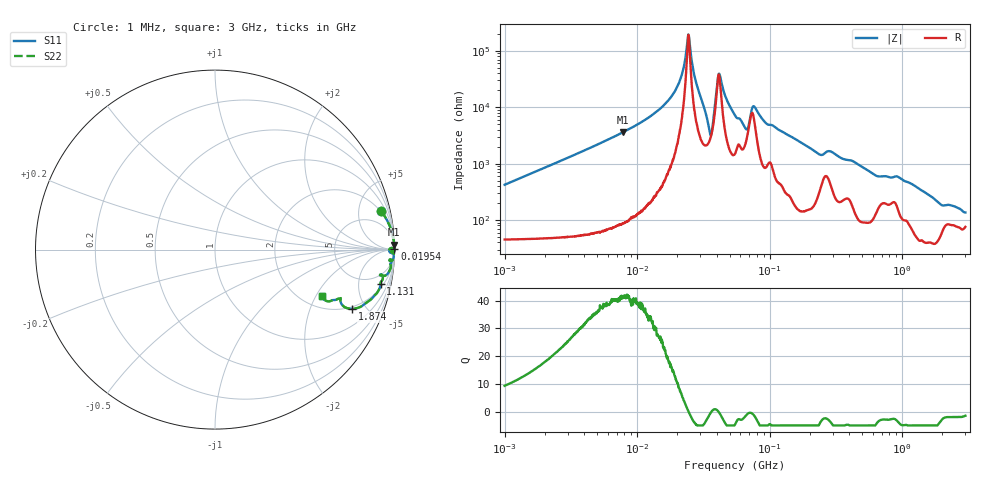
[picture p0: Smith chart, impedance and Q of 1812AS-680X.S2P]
!s-Parameter Generated by FASTRON Sdn. Bhd.
!FASTRON P/N : 1812AS-680X
!Keysight Technologies,E4991B,MY54100416,A.01.15
!Date created: Mon Oct 16 10:20:13 2023
!Version  : Rev00 Mon Oct 16 10:20:13 2023
!Data & Calibration Information:
!Freq	S11	S21	S12	S22
!PortZ  Port1:50+j0  Port2:50+j0
!When reading, reference impedance value at option line is always used.
! Remarks : This data is being provided solely for informational purposes.
# Hz S dB R 50
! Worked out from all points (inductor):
!   1601 points, 1 MHz to 3 GHz, reference 50 ohm
!   read as one part in series: L = 66.6 uH near 1.041 MHz
!   highest Q = 41.6 at 7.82 MHz (marker M1), where L = 73.1 uH
!   self-resonance near 24.35 MHz
!   S11 on the Smith chart (normalised r, x): 1 MHz: 1.90, +8.39; 19.54 MHz: open; 1.131 GHz: 2.64, -9.02; 1.874 GHz: 1.87, -3.99; 3 GHz: 2.51, -2.26
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1000000  -0.44 12.9  -12.95 -70.9  -12.95 -70.9  -0.44 12.9
3804036  -0.03 3.5  -24.26 -84.6  -24.26 -84.6  -0.03 3.5
7819618  -0.01 1.6  -31.12 -87.0  -31.12 -87.0  -0.01 1.6
1.447069e7  -0.00 0.6  -38.93 -87.2  -38.93 -87.2  -0.00 0.6
1.953805e7  -0.00 0.3  -46.19 -84.8  -46.19 -84.8  -0.00 0.3
2.181181e7  -0.00 0.1  -51.78 -80.1  -51.78 -80.1  -0.00 0.1
2.37485e7  -0.00 0.0  -61.82 -53.7  -61.82 -53.7  -0.00 0.0
2.447233e7  -0.00 -0.0  -65.59 5.7  -65.59 5.7  -0.00 -0.0
2.759511e7  -0.01 -0.2  -49.47 77.0  -49.47 77.0  -0.01 -0.2
3.543987e7  -0.19 -1.0  -31.05 39.6  -31.05 39.6  -0.19 -1.0
3.688738e7  -0.20 0.4  -32.37 -17.8  -32.37 -17.8  -0.20 0.4
4.016263e7  -0.03 0.1  -48.11 -26.8  -48.11 -26.8  -0.03 0.1
4.180303e7  -0.02 -0.1  -51.79 27.6  -51.79 27.6  -0.02 -0.1
5.477226e7  -0.03 -0.8  -37.14 77.1  -37.14 77.1  -0.03 -0.8
6.690963e7  -0.14 -1.1  -32.28 47.8  -32.28 47.8  -0.14 -1.1
7.697298e7  -0.04 -0.5  -40.17 58.3  -40.17 58.3  -0.04 -0.5
9.497575e7  -0.03 -1.1  -34.16 78.9  -34.16 78.9  -0.03 -1.1
2.083556e8  -0.06 -3.2  -25.14 81.7  -25.14 81.7  -0.06 -3.2
7.925923e8  -0.58 -8.8  -15.79 62.3  -15.79 62.3  -0.58 -8.8
1.130699e9  -0.51 -11.7  -13.74 68.0  -13.74 68.0  -0.51 -11.7
1.874306e9  -1.61 -23.4  -7.81 54.2  -7.81 54.2  -1.61 -23.4
3e9  -3.72 -23.5  -6.40 32.8  -6.40 32.8  -3.72 -23.5
